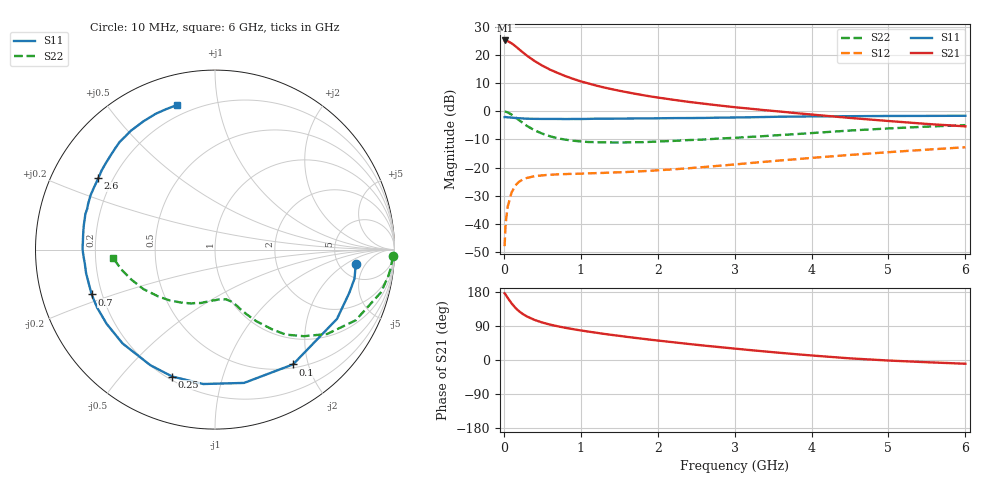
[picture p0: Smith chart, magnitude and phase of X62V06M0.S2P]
! SIEMENS Small Signal Semiconductors
! BFP193W
! Si NPN RF Bipolar Junction Transistor in SOT343
! VCE = 2 V  IC = 6 mA
! Common Emitter S-Parameters:  April 1994
# GHz  S  MA  R  50
!  f  S11  S21  S12  S22
! GHz  MAG  ANG  MAG  ANG  MAG  ANG  MAG  ANG
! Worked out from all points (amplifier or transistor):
!   40 points, 10 MHz to 6 GHz, reference 50 ohm
!   highest |S21| = 25.2 dB at 20 MHz (marker M1)
!   |S21| within 3 dB of that: start of sweep to 192.3 MHz
!   unconditionally stable (mu >= 1): 1.557 GHz to 4.579 GHz
!   at 200 MHz: K = 0.16, MSG = 23.5 dB, |S12| = -25.0 dB
!   at 1.5 GHz: K = 0.98, MSG = 14.5 dB, |S12| = -21.7 dB
!   at 6 GHz: K = 0.94, MSG = 3.7 dB, |S12| = -12.8 dB
!   lowest NFmin = 1.20 dB at 450 MHz
!   S11 on the Smith chart (normalised r, x): 10 MHz: 7.13, -3.05; 100 MHz: 0.55, -1.76; 250 MHz: 0.22, -0.70; 700 MHz: 0.16, -0.17; 2.6 GHz: 0.15, +0.28; 6 GHz: 0.14, +0.76
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0.01  0.7885 -5.9  18.14 176.0  0.004 85.4  0.9919 -2.2
0.02  0.7939 -11.8  18.17 173.5  0.0083 82.9  0.9846 -6.1
0.05  0.7817 -29.6  17.69 164.0  0.0201 75.7  0.9545 -14.5
0.1  0.7734 -55.8  16.19 149.7  0.0359 63.4  0.8771 -26.7
0.15  0.7602 -77.7  14.41 137.6  0.0481 53.2  0.7817 -37.0
0.2  0.7518 -95.0  12.6 128.2  0.0561 45.8  0.6908 -44.3
0.25  0.7463 -108.6  11.08 120.9  0.0618 39.7  0.6166 -50.2
0.3  0.738 -119.2  9.751 114.9  0.0654 35.7  0.5497 -54.2
0.4  0.7339 -134.6  7.824 105.7  0.0702 30.0  0.4595 -60.1
0.5  0.7318 -145.6  6.49 98.9  0.0726 27.1  0.4003 -64.0
0.6  0.732 -153.7  5.507 93.4  0.0744 25.0  0.3598 -67.0
0.7  0.7313 -160.0  4.809 89.0  0.0756 24.2  0.3314 -69.1
0.9  0.7301 -169.6  3.78 81.4  0.0772 23.6  0.2999 -73.3
1.1  0.7334 -177.0  3.129 74.9  0.079 24.1  0.2844 -77.2
1.3  0.7373 176.8  2.656 69.0  0.0804 25.6  0.2801 -81.3
1.6  0.7437 169.2  2.184 61.1  0.0833 28.4  0.2796 -87.4
2.2  0.7566 156.4  1.605 46.9  0.0928 34.4  0.2971 -100.5
2.6  0.7619 148.6  1.365 38.1  0.1021 37.9  0.3148 -109.5
3.2  0.7829 138.1  1.113 26.2  0.1201 41.1  0.3505 -122.7
4.5  0.8185 119.1  0.762 4.3  0.1675 40.7  0.455 -151.0
5.5  0.8283 109.4  0.596 -5.9  0.208 36.7  0.5339 -168.1
6  0.8327 104.9  0.54 -9.9  0.2295 34.3  0.5677 -175.0
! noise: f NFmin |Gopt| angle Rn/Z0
0.45  1.2  0.25  114  0.13
0.9  1.25  0.37  150  0.12
1.8  2  0.55  -158  0.12
